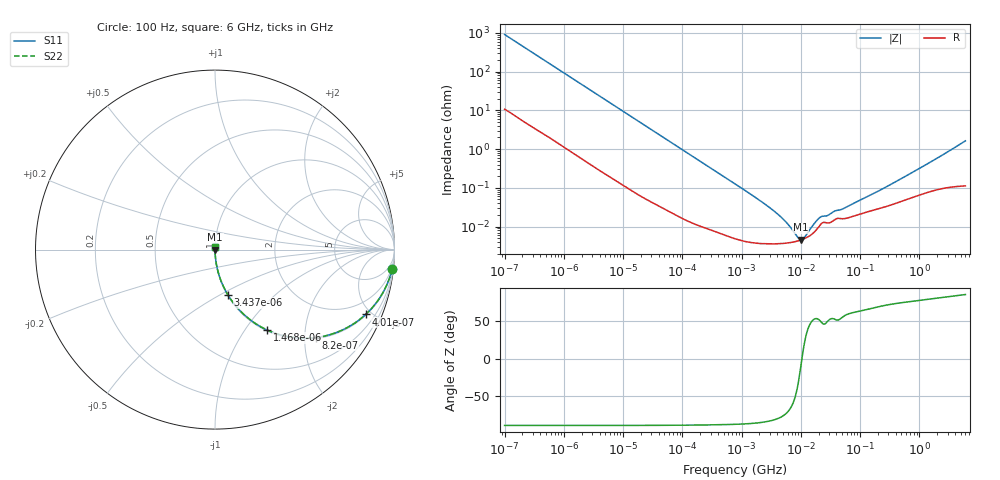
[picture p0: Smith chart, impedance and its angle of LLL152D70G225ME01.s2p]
!Murata Part Number: LLL152D70G225ME01
!These Parameters are Measured in Series Mode Connection
!Data Generated on Jan 08, 2026
!  o--ll--o
!Port1  Port2
!  o------o
!Operation Temp=25[degC], DC Bias Voltage=0[V]
!Freq. Start=100[Hz] Stop=6[GHz] 401[Steps]
# Hz S RI R 50
!Freq.(Hz) S11(Real) S11(Imag) S21(Real) S21(Imag) S12(Real) S12(Imag) S22(Real) S22(Imag)
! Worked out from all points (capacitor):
!   401 points, 100 Hz to 6 GHz, reference 50 ohm
!   read as one part in series: C = 1.73 uF near 109 Hz
!   lowest |Z| = 4.55 mohm at 9.942 MHz (marker M1)
!   series resonance near 10.44 MHz, so ESL is about 130 pH
!   S11 on the Smith chart (normalised r, x): 100 Hz: 1, -18; 401 Hz: 1.06, -4.62; 820 Hz: 1.03, -2.27; 1.468 kHz: 1.02, -1.27; 3.437 kHz: 1.01, -0.55; 6 GHz: 1.00, +0.03
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100  0.987 -0.1076  0.013 0.1076  0.013 0.1076  0.987 -0.1076
224  0.9419 -0.2281  0.0581 0.2281  0.0581 0.2281  0.9419 -0.2281
401  0.8393 -0.3613  0.1607 0.3613  0.1607 0.3613  0.8393 -0.3613
820  0.5623 -0.4901  0.4377 0.4901  0.4377 0.4901  0.5623 -0.4901
1468  0.291 -0.4483  0.709 0.4483  0.709 0.4483  0.291 -0.4483
2008  0.1819 -0.3798  0.8181 0.3798  0.8181 0.3798  0.1819 -0.3798
3437  0.0724 -0.2532  0.9276 0.2532  0.9276 0.2532  0.0724 -0.2532
9626  0.0108 -0.0974  0.9892 0.0974  0.9892 0.0974  0.0108 -0.0974
40335  0.000902 -0.0237  0.9991 0.0237  0.9991 0.0237  0.000902 -0.0237
774597  4.99e-05 -0.00127  1 0.00127  1 0.00127  4.99e-05 -0.00127
3103719  3.56e-05 -0.000291  1 0.000291  1 0.000291  3.56e-05 -0.000291
6353432  3.81e-05 -9.83e-05  1 9.83e-05  1 9.83e-05  3.81e-05 -9.83e-05
7266822  3.94e-05 -7.03e-05  1 7.03e-05  1 7.03e-05  3.94e-05 -7.03e-05
9941735  4.46e-05 -9.2e-06  1 9.2e-06  1 9.2e-06  4.46e-05 -9.2e-06
1.422411e7  5.8e-05 6.03e-05  0.9999 -6.03e-05  0.9999 -6.03e-05  5.8e-05 6.03e-05
1.555665e7  6.41e-05 7.85e-05  0.9999 -7.85e-05  0.9999 -7.85e-05  6.41e-05 7.85e-05
2.225763e7  0.000119 0.000136  0.9999 -0.000136  0.9999 -0.000136  0.000119 0.000136
2.784235e7  0.000124 0.000145  0.9999 -0.000145  0.9999 -0.000145  0.000124 0.000145
3.80911e7  0.000154 0.000202  0.9998 -0.000202  0.9998 -0.000202  0.000154 0.000202
5.211241e7  0.000159 0.000241  0.9998 -0.000241  0.9998 -0.000241  0.000159 0.000241
3.124326e8  0.000349 0.00112  0.9997 -0.00112  0.9997 -0.00112  0.000349 0.00112
6e9  0.00138 0.0163  0.9986 -0.0163  0.9986 -0.0163  0.00138 0.0163
